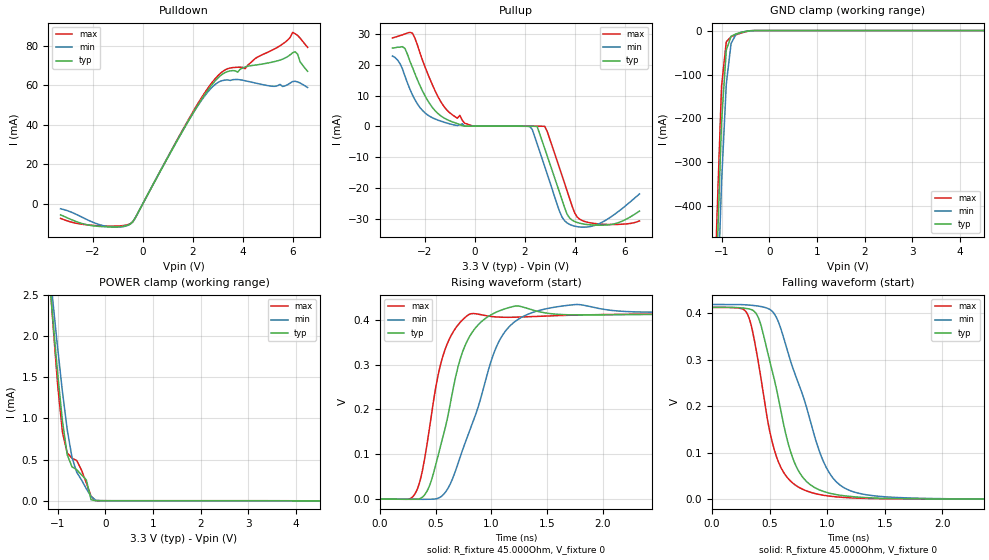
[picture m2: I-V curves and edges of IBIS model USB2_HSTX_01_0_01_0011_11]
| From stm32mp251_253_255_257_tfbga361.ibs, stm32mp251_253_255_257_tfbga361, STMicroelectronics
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[Model] USB2_HSTX_01_0_01_0011_11
Model_type   Output
Polarity   Non-Inverting
Enable   Active-High
C_comp   8.036pF   7.631pF   8.569pF
Vmeas = 200.000mV
Vref = 200.000mV
Rref = 45Ohms
Cref = 0pF
[Model Spec]
Vmeas   200.000mV   200.000mV   200.000mV
Vref   200.000mV   200.000mV   200.000mV
| This model is not intended for timing simulations.
| Warnings about Cref, Vref & Rref can be ignored
[Temperature Range]   25.000   125.000   -40.000
[Voltage Range]   3.300V   3.070V   3.630V
[GND Clamp Reference]   0.00V   0.00V   0.00V
[Pulldown Reference]   0.00V   0.00V   0.00V
[POWER Clamp Reference]   3.300V   3.070V   3.630V
[Pullup Reference]   3.300V   3.070V   3.630V
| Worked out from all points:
|   slope of the pulldown table from 0 to 0.495 V, typ, clamps not added: 42.6 ohm
|   GND clamp passes 1 mA (typ) near -0.43 V on its own axis
|   POWER clamp passes 1 mA (typ) near -0.91 V on its own axis
|   rising waveform, R_fixture 45.000Ohm, V_fixture 0: 20-80 % time 238ps typ, 332ps min, 184ps max; typ from 0 V to 0.413 V
|   falling waveform, R_fixture 45.000Ohm, V_fixture 0: 20-80 % time 242ps typ, 327ps min, 196ps max; typ from 0.413 V to 0 V
[GND Clamp]
-3.3V     -11.02A    -10.62A    -11.32A
-1.2V     -931.6mA   -1.049A    -855.7mA
-1.1V     -533.1mA   -671.7mA   -440.2mA
-1V       -209.4mA   -347mA     -127.3mA
-900mV    -44.44mA   -121.7mA   -25.6mA
-800mV    -13.15mA   -29.48mA   -14.15mA
-700mV    -7.742mA   -9.125mA   -9.769mA
-500mV    -2.127mA   -1.981mA   -2.894mA
-300mV    -19.47uA   -62.22uA   -13.77uA
6.6V      10.37uA    26.59uA    21.05uA
[Power Clamp]
-3.3V     3.206A     2.175A     4.855A
-1.2V     2.88mA     3.008mA    2.969mA
-1.1V     2.195mA    2.419mA    2.156mA
-1V       1.545mA    1.852mA    1.406mA
-900mV    967.9uA    1.324mA    831.4uA
-800mV    558.4uA    864.6uA    580.3uA
-700mV    412uA      525.9uA    517uA
-600mV    376.6uA    345uA      488.5uA
-400mV    254.2uA    146.6uA    216.8uA
-300mV    11.21uA    52.87uA    53.51uA
-100mV    94.77nA    985nA      361.1nA
6.6V      -2.736uA   -5.18uA    -2.975uA
[Pulldown]
-3.3V     -5.671mA   -2.581mA   -7.449mA
-1.6V     -11.64mA   -11.09mA   -11.31mA
-500mV    -10.25mA   -10.32mA   -10.1mA
1.9V      43.42mA    43.46mA    44.13mA
2.9V      62.15mA    60.37mA    63.26mA
3.4V      66.87mA    62.63mA    68.29mA
4.1V      69.19mA    62.19mA    68.26mA
4.5V      70.11mA    61.06mA    73.4mA
5.6V      73.12mA    59.29mA    80.76mA
6V        76.33mA    61.79mA    86.69mA
6.1V      76.87mA    61.92mA    85.99mA
6.6V      66.99mA    58.79mA    79.1mA
[Pullup]
-3.3V     25.41mA    22.86mA    28.69mA
-2.8V     25.3mA     16.38mA    30mA
-2.5V     19.22mA    10.28mA    30.27mA
-1.2V     2.602mA    1.31mA     6.11mA
-100mV    93.8uA     82.61uA    220.4uA
2.2V      68.66uA    -28.24uA   104.8uA
2.5V      -41.4uA    -5.658mA   83.47uA
2.9V      -9.472mA   -15.37mA   -1.563mA
3.5V      -23.92mA   -29.44mA   -16.02mA
3.8V      -29.68mA   -31.75mA   -23.35mA
4.4V      -31.68mA   -32.65mA   -30.79mA
6.6V      -27.44mA   -21.87mA   -30.63mA
[Ramp]
R_load=45.000Ohm
dV/dt_r   624.171mV/1.100ns  592.503mV/1.145ns  677.762mV/1.005ns
dV/dt_f   626.381mV/265.000ps  595.438mV/350.000ps  679.594mV/225.000ps
[Rising waveform]
R_fixture=45.000Ohm
V_fixture=0
0s        452.3nV    3.134uV    468nV
330ps     -200.2uV   -412.7uV   19.76mV
440ps     27.56mV    -306.8uV   152mV
590ps     163.9mV    16.52mV    338.2mV
700ps     295.1mV    79.65mV    388.5mV
800ps     361.1mV    149.4mV    411.9mV
1.04ns    416.5mV    337mV      406.3mV
1.21ns    430.3mV    395.7mV    405.6mV
1.77ns    410.7mV    434mV      410.5mV
9.9ns     413.1mV    419.1mV    412.8mV
[Falling waveform]
R_fixture=45.000Ohm
V_fixture=0
0s        412.6mV    418.6mV    412.3mV
310ps     409.6mV    417.6mV    396.7mV
410ps     385.7mV    414.9mV    283.8mV
540ps     258.8mV    398.9mV    107.4mV
650ps     130.9mV    323.5mV    48.1mV
720ps     76.96mV    269.7mV    31.34mV
960ps     17.67mV    85.68mV    9.073mV
1.17ns    6.948mV    21.88mV    3.654mV
1.66ns    1.332mV    3.373mV    908uV
9.9ns     13.74uV    31.08uV    3.863uV
